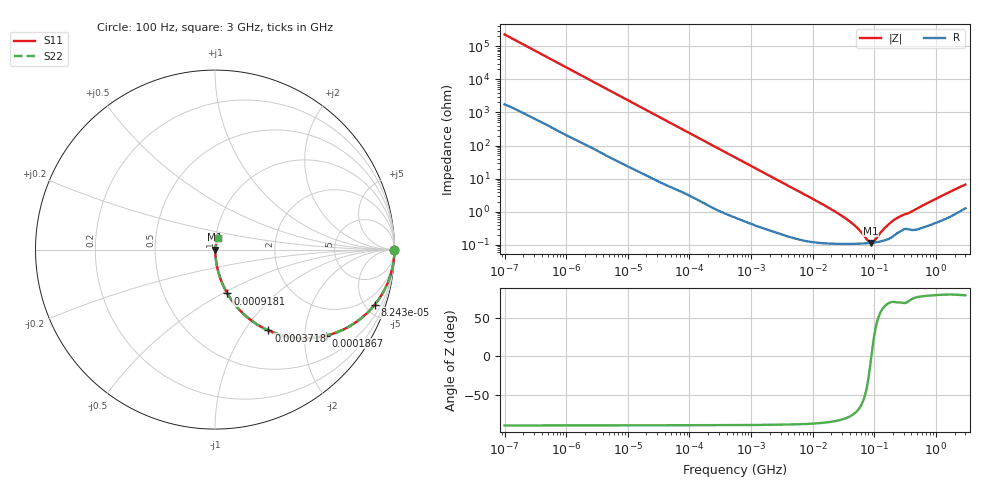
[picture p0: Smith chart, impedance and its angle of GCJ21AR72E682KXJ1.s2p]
!Murata Part Number: GCJ21AR72E682KXJ1
!These Parameters are Measured in Series Mode Connection
!Data Generated on Mar 13, 2026
!  o--ll--o
!Port1  Port2
!  o------o
!Operation Temp=25[degC], DC Bias Voltage=0[V]
!Freq. Start=100[Hz] Stop=3[GHz] 401[Steps]
# Hz S RI R 50
!Freq.(Hz) S11(Real) S11(Imag) S21(Real) S21(Imag) S12(Real) S12(Imag) S22(Real) S22(Imag)
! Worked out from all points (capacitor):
!   401 points, 100 Hz to 3 GHz, reference 50 ohm
!   read as one part in series: C = 6.98 nF near 109 Hz
!   lowest |Z| = 114 mohm at 87.97 MHz (marker M1)
!   series resonance near 89.42 MHz, so ESL is about 450 pH
!   S11 on the Smith chart (normalised r, x): 100 Hz: open; 82.43 kHz: 1.07, -5.76; 186.7 kHz: 1.03, -2.56; 371.8 kHz: 1.02, -1.29; 918.1 kHz: 1.01, -0.53; 3 GHz: 1.03, +0.13
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100  1 -0.000439  3.6e-06 0.000439  3.6e-06 0.000439  1 -0.000439
1788  0.9999 -0.00772  0.000131 0.00772  0.000131 0.00772  0.9999 -0.00772
10443  0.9976 -0.0445  0.00243 0.0445  0.00243 0.0445  0.9976 -0.0445
31977  0.9806 -0.1328  0.0194 0.1328  0.0194 0.1328  0.9806 -0.1328
82428  0.8894 -0.3073  0.1106 0.3073  0.1106 0.3073  0.8894 -0.3073
121426  0.7908 -0.4003  0.2092 0.4003  0.2092 0.4003  0.7908 -0.4003
186741  0.6197 -0.4791  0.3803 0.4791  0.3803 0.4791  0.6197 -0.4791
263501  0.4534 -0.4913  0.5466 0.4913  0.5466 0.4913  0.4534 -0.4913
371814  0.2971 -0.4502  0.7029 0.4502  0.7029 0.4502  0.2971 -0.4502
547723  0.1659 -0.3645  0.8341 0.3645  0.8341 0.3645  0.1659 -0.3645
918067  0.0687 -0.2444  0.9313 0.2444  0.9313 0.2444  0.0687 -0.2444
2470636  0.012 -0.0974  0.988 0.0974  0.988 0.0974  0.012 -0.0974
9794414  0.00182 -0.0249  0.9982 0.0249  0.9982 0.0249  0.00182 -0.0249
3.71925e7  0.00109 -0.0055  0.9989 0.0055  0.9989 0.0055  0.00109 -0.0055
5.248048e7  0.00108 -0.00309  0.9989 0.00309  0.9989 0.00309  0.00108 -0.00309
7.730952e7  0.00112 -0.000807  0.9989 0.000807  0.9989 0.000807  0.00112 -0.000807
8.79653e7  0.00114 -8.95e-05  0.9989 8.95e-05  0.9989 8.95e-05  0.00114 -8.95e-05
1.000898e8  0.00117 0.000627  0.9988 -0.000627  0.9988 -0.000627  0.00117 0.000627
1.352818e8  0.00131 0.00237  0.9987 -0.00237  0.9987 -0.00237  0.00131 0.00237
1.751444e8  0.00155 0.00404  0.9985 -0.00404  0.9985 -0.00404  0.00155 0.00404
2.693545e8  0.00263 0.00693  0.9974 -0.00693  0.9974 -0.00693  0.00263 0.00693
3e9  0.0165 0.0629  0.9835 -0.0629  0.9835 -0.0629  0.0165 0.0629
